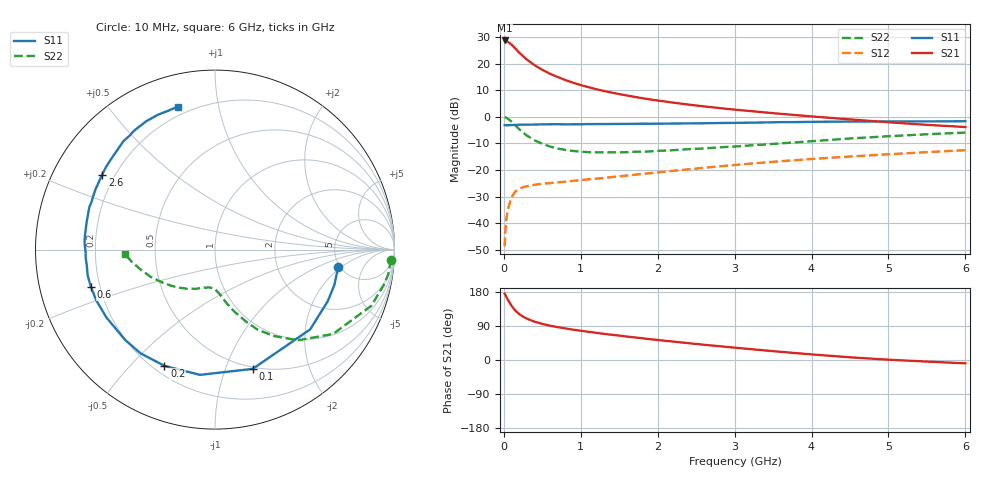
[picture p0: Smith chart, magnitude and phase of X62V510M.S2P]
! SIEMENS Small Signal Semiconductors
! BFP193W
! Si NPN RF Bipolar Junction Transistor in SOT343
! VCE = 2.5 V  IC = 10 mA
! Common Emitter S-Parameters:  April 1994
# GHz  S  MA  R  50
!  f  S11  S21  S12  S22
! GHz  MAG  ANG  MAG  ANG  MAG  ANG  MAG  ANG
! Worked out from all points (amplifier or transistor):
!   40 points, 10 MHz to 6 GHz, reference 50 ohm
!   highest |S21| = 28.7 dB at 10 MHz (marker M1)
!   |S21| within 3 dB of that: start of sweep to 148.1 MHz
!   unconditionally stable (mu >= 1): 1.274 GHz to 4.12 GHz
!   at 200 MHz: K = 0.22, MSG = 25.6 dB, |S12| = -27.2 dB
!   at 1.5 GHz: K = 1.07, MAG = 13.8 dB, |S12| = -22.4 dB
!   at 6 GHz: K = 0.93, MSG = 4.3 dB, |S12| = -12.6 dB
!   lowest NFmin = 1.30 dB at 450 MHz
!   S11 on the Smith chart (normalised r, x): 10 MHz: 4.81, -1.81; 100 MHz: 0.48, -1.25; 200 MHz: 0.24, -0.63; 600 MHz: 0.16, -0.14; 2.6 GHz: 0.15, +0.30; 6 GHz: 0.15, +0.76
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0.01  0.6931 -8.1  27.1 175.0  0.0037 87.1  0.9823 -3.3
0.02  0.6937 -16.4  27.04 171.6  0.0074 81.6  0.9744 -8.3
0.03  0.6908 -24.6  26.84 167.6  0.0111 78.9  0.9596 -12.1
0.05  0.692 -40.0  25.84 159.7  0.0178 72.5  0.9251 -19.8
0.1  0.6968 -72.5  22.54 143.1  0.0308 58.2  0.8086 -35.5
0.15  0.7028 -96.8  19.06 130.2  0.0394 48.3  0.6849 -47.6
0.2  0.7063 -113.5  16.02 121.1  0.0438 42.0  0.5827 -55.7
0.25  0.7114 -125.7  13.73 114.3  0.0474 37.4  0.5062 -61.9
0.3  0.7099 -134.9  11.84 109.1  0.0495 34.8  0.4422 -66.3
0.4  0.7135 -148.0  9.293 101.1  0.0526 31.8  0.3605 -72.8
0.5  0.7193 -156.7  7.609 95.2  0.0551 31.1  0.3098 -77.3
0.6  0.7219 -163.3  6.412 90.6  0.0567 31.0  0.2756 -80.9
0.8  0.7198 -172.8  4.88 83.3  0.0602 32.6  0.2381 -86.0
1.1  0.7274 177.5  3.599 74.4  0.0667 36.0  0.2157 -92.5
1.3  0.7288 172.1  3.05 69.0  0.0707 38.3  0.2135 -96.4
1.6  0.7334 165.3  2.504 61.8  0.0786 41.3  0.216 -101.8
2.2  0.7453 153.5  1.842 48.6  0.0963 44.9  0.2354 -113.3
2.6  0.7545 146.4  1.565 40.3  0.1097 45.9  0.2537 -121.0
3.2  0.7726 136.3  1.28 28.8  0.1312 45.7  0.2888 -132.5
4.5  0.8113 118.2  0.891 7.1  0.1787 41.0  0.3901 -157.2
5.5  0.8159 108.9  0.703 -4.2  0.216 35.9  0.4682 -171.6
6  0.8234 104.5  0.641 -8.8  0.2356 33.5  0.5036 -177.4
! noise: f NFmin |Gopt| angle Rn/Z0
0.45  1.3  0.22  143  0.11
0.9  1.3  0.34  160  0.11
1.8  2.05  0.54  -153  0.14
